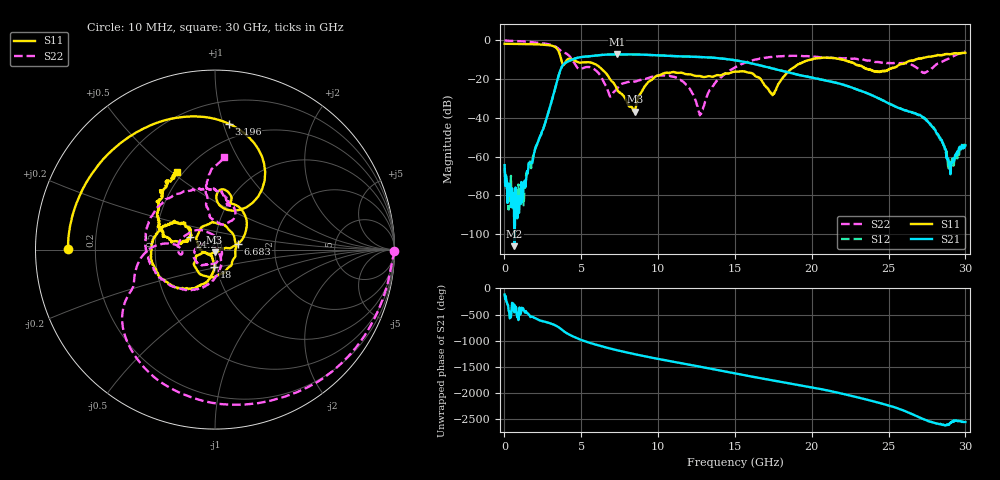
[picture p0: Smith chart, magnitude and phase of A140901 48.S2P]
!  2-Port S-parameters saved by WinCal
! VAR MeasName=S-Parameters (CALIBRATED_DATA) read from VNA (N5244A)
! VAR MeasDate=11/3/2014 9:34:22 AM
! VAR NAME=A140901 48
! VAR FILENAME=A140901 48.S2P
! VAR DATE=11/3/2014 9:34:22 AM
! VAR PHYS_PORTS=1,2
# Hz S RI R 50
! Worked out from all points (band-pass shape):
!   801 points, 10 MHz to 30 GHz, reference 50 ohm
!   highest |S21| = -7.17 dB at 7.32 GHz (marker M1); lowest = -106.3 dB at 647.3 MHz (marker M2)
!   |S21| within 3 dB of the highest: 4.329 GHz to 14.93 GHz (10.6 GHz wide, 110 % of centre)
!   lowest |S11| = -36.8 dB at 8.482 GHz (marker M3), VSWR 1.03, Z = 49.8 - j1.42 ohm
!   |S11| at or under -10 dB: 3.701 GHz to 4.08 GHz (379.2 MHz wide, 9.75 % of centre); 4.463 GHz to 19.91 GHz (15.45 GHz wide, 127 % of centre); 22.1 GHz to 26.72 GHz (4.628 GHz wide, 19 % of centre)
!   |S22| runs from -38.7 to 0.0 dB; largest |S21 - S12| = 0.003
!   S11 on the Smith chart (normalised r, x): 10 MHz: 0.10, +0.00; 3.196 GHz: 0.37, +1.04; 6.683 GHz: 1.29, +0.08; 18 GHz: 0.98, -0.19; 24.26 GHz: 0.75, +0.11; 30 GHz: 0.47, +0.52
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1e7  -0.8198 0.00171  -0.000261 -0.000539  0.000417 -0.000277  0.9983 -0.00793
6.472875e8  -0.7885 0.2089  -4.14e-07 -4.81e-06  -3.78e-05 -5.37e-06  0.8836 -0.3924
1.2096e9  -0.7133 0.3801  8.02e-05 -2.28e-05  2.39e-05 -8.23e-05  0.6717 -0.6628
3.196438e9  0.0754 0.7021  0.035 0.021  0.0349 0.0207  -0.4615 -0.567
3.833725e9  0.0697 0.2211  -0.00178 -0.239  -0.00118 -0.2379  -0.4528 -0.1952
4.396038e9  0.0767 0.3169  -0.3163 0.0343  -0.3159 0.0332  -0.3238 0.0243
5.033325e9  0.0827 0.2543  -0.0262 0.3719  -0.0266 0.3717  -0.1852 -0.0261
6.682775e9  0.1262 0.0325  0.2652 -0.3401  0.2654 -0.3394  0.0221 0.0516
7.320062e9  0.0556 0.00756  -0.0684 -0.4327  -0.0676 -0.4319  0.0251 -0.0495
8.482175e9  -0.00215 -0.0143  -0.4319 -0.0353  -0.4316 -0.0362  -0.036 -0.0781
1.001916e10  -0.1024 0.0721  -0.0252 0.4113  -0.025 0.4099  -0.0989 -0.0758
1.17061e10  0.07 0.1199  0.3845 0.0106  0.3845 0.0112  -0.0732 0.0302
1.275575e10  0.1199 0.0157  0.2113 -0.3058  0.2117 -0.3056  0.00992 0.00838
1.5005e10  -0.0203 -0.1533  -0.3068 0.00894  -0.3071 0.00927  -0.0406 -0.1965
1.74042e10  -0.0257 -0.0337  0.1287 0.1394  0.1284 0.141  -0.3714 -0.0512
1.8004e10  -0.00359 -0.0952  0.1588 0.0471  0.1601 0.048  -0.386 0.049
2.002832e10  -0.2722 -0.1784  0.000946 -0.109  0.000959 -0.11  -0.2406 0.2941
2.426441e10  -0.138 0.0701  0.0318 -0.00832  0.0318 -0.00849  0.0737 0.2658
2.501416e10  -0.1665 0.0457  0.00583 -0.0227  0.00584 -0.0229  0.0706 0.2533
2.745085e10  -0.3191 0.1865  0.00876 0.000627  0.009 0.000361  0.0166 0.1498
2.902532e10  -0.2821 0.3385  0.000225 -0.000265  0.000405 -0.000576  -0.0494 0.3542
3e10  -0.2091 0.4305  0.00167 -0.00102  0.0017 -0.000976  0.0517 0.5175
